(* Logix 5000 AddOnInstructionDefinition export NTEC_VerifyLimits; software revision ? *)

TYPE NTEC_Axis :   // NTEC Axis:
STRUCT
   StatDriveCommsOK : BOOL;   // Drive is communicating over ENET IP
   StatServoActionStatus : BOOL;   // Motion is enabled and holding position under power.
   StatDriveWarning : BOOL;   // Drive has a Warning
   StatDriveFault : BOOL;   // Drive is Faulted
   StatMotion_AtTarget : BOOL;   // Motion Target Reached
   StatMotion_FollowingError : BOOL;   // Following Error Fault
   StatMotion_LimitExceeded : BOOL;   // Speed or Position Limit Exceeded
   StatMotion_Halt : BOOL;   // Motor is in Halt, still powered on
   StatQuckStop : BOOL;   // Motor is powered off in Quick Stop
   StatMotion_Homed : BOOL;   // Motion Coordinate System Homed
   StatNewCmdToggle : BOOL;   // Bit toggles after new command accepted
   StatCommandError : BOOL;   // Last Command has an Error
   StatCommandErrorCode : DINT;   // Command Error Code
   StatDriveFaultCode : DINT;   // Drive Fault Code
   StatDriveWarningCode : DINT;   // Drive Warning Code
   StatResettingFault : BOOL;   // In fault reset sequence
   StatReadResponse : DINT;   // Response from a Read CMD
   CMD_IP : BOOL;   // Command is In Process
   CMD_DN : BOOL;   // Command is Done
   CMD_ERR : BOOL;   // Command Error during Comms send to Drive
   PDI_CMD : NTEC_PDI_CMD;   // Commands from AOIs
   PDI_Status : NTEC_PDI_Status;   // Status from Drive out to AOIs
   DriveLimits : NTEC_LimitsInDrive;   // Limits read from Drive
END_STRUCT
END_TYPE

TYPE NTEC_LimitsInDrive :   // These are the limits read from the Drive
STRUCT
   PositionLimitMin : DINT;   // Minimum Allowed Position Target (607Bh:1)
   PositionLimitMax : DINT;   // Maximum Allowed Position Target (607Bh:2)
   SoftPositionLimitMin : DINT;   // Minimum Allowed Position (607Dh:1)
   SoftPositionLimitMax : DINT;   // Minimum Allowed Position (607Dh:2)
   VelocityLimitMin : DINT;   // Maximum Allowed Velocity Target negative direction
   VelocityLimitMax : DINT;   // Maximum Allowed Velocity Target positive direction (607Fh)
   MotorSpeedMin : DINT;   // Maximum motor speed in negative direction
   MotorSpeedMax : DINT;   // Maximum motor speed setting in positive direction (6080h)
   AccelLimitMax : DINT;   // Maximum Allowed Accel Target (60C5h)
   DecelLimitMax : DINT;   // Maximum Allowed Decel Target (60C6h)
   PositionWindowNeg : DINT;   // Position Window - negative direction for At Target (6067h)
   PositionWindowPos : DINT;   // Position Window -positive direction for At Target (+/- this value) (6067h)
   VelocityWindowNeg : DINT;   // Velocity Window - negative side for At Target (+/- this value) (606Dh)
   VelocityWindowPos : DINT;   // Velocity Window - positive side for At Target (+/- this value) (606Dh)
   TorqueMaxNegDir : DINT;   // Maximum Torque Target negative direction (0.1% of motor rated current 2031h) (6072h)
   TorqueMaxPosDir : DINT;   // Maximum Torque Target positive direction (0.1% of motor rated current 2031h) (6072h)
   CurrentMaxNegDir : DINT;   // Maximum Current Target negative direction (in 0.1% of rated setting 2031h) (6073h)
   CurrentMaxPosDir : DINT;   // Maximum Current Target positive direction (in 0.1% of rated setting 2031h) (6073h)
END_STRUCT
END_TYPE

TYPE NTEC_PDI_CMD :   // PDI Command Bytes
STRUCT
   SetValue1 : DINT;
   SetValue2 : INT;
   SetValue3 : SINT;
   CMD : SINT;
   DigitalOutputs : DINT;
   NanoJ_Input1 : DINT;
   Trig : BOOL;   // Trigger the Command
   Halt : BOOL;   // Command a HALT
   QuickStop : BOOL;   // Command a QuickStop
END_STRUCT
END_TYPE

TYPE NTEC_PDI_Status :   // PDI Status Bytes
STRUCT
   Status : INT;
   ErrorCode : INT;
   ReturnValue : DINT;
   PositionActualValue : DINT;
   VelocityActualValue : DINT;
   DigitalInputs : DINT;
   TorqueActualValue : INT;
   AnalogInput1 : INT;
   FollowingError : DINT;
   NanoJ_Output1 : DINT;
END_STRUCT
END_TYPE

ADD_ON_INSTRUCTION NTEC_READ   (* revision 1.6, vendor Third Coast Automation, Nashville, TN, ExecutePrescan, ExecuteEnableInFalse *)
// READ instruction reads the value of  one object from the Drive.  Enter the target object's index and sub-index (typically 16#xxxx hex values).
// Revision note:
// Release Aug 27, 2024, update CPS instructions LEN
// Help:
// AOI written by:
// Tim Cochran
// Third Coast Automation
// Nashville, TN
// MAS ERR_Codes:
// 2: Input parameter range error – review and fix input parameters.
// 3: Command Error response from the Drive after command sent.
// 10: Communications Failed to Drive.
// 11: Drive Fault during this AOIs command sequence.
// 12: Quick Stop triggered by software outside of this AOI.
// 13: Command Error response from the Drive.
// 14: Enable input changed to False during sequence due to Drive Fault or Offline.
VAR_IN_OUT
   NTEC_Axis : NTEC_Axis; {required}   // NTEC Axis Tag
END_VAR
VAR_INPUT
   Index : DINT; {required}   // Index
   SubIndex : DINT; {required}   // Sub-Index
END_VAR
VAR_OUTPUT
   EN : BOOL; {visible}   // Enabled
   DN : BOOL; {visible}   // Successfully Done
   Read_Value : DINT; {visible}   // Value Read from Drive
   ERR : BOOL; {visible}   // Instruction Error
   ERR_Code : DINT; {access Read Only, visible}   // Instruction Error Code
END_VAR
VAR
   State : DINT; {access None}
   Enable : BOOL; {access None}
   InputRangesOK : BOOL; {access None}
   local_SubIndex : DINT; {access None}
   local_Index : DINT; {access None}
   tmr_Verify : TIMER := (PRE := 20); {access None}
END_VAR

ROUTINE EnableInFalse   (* ladder *)
// Enable In False Routine
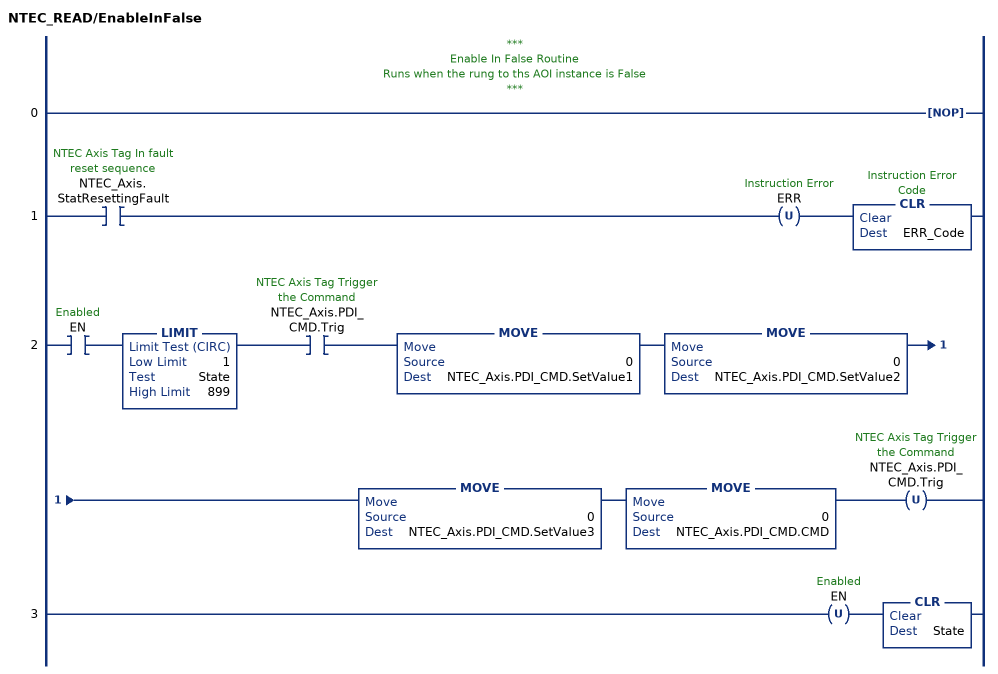
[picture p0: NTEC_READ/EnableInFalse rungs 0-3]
   // ***
   // Enable In False Routine
   // Runs when the rung to ths AOI instance is False
   // ***
   0: NOP();
   1: XIC(NTEC_Axis.StatResettingFault)OTU(ERR)CLR(ERR_Code);
   2: XIC(EN)LIMIT(1,State,899)XIC(NTEC_Axis.PDI_CMD.Trig)MOVE(0,NTEC_Axis.PDI_CMD.SetValue1)MOVE(0,NTEC_Axis.PDI_CMD.SetValue2)MOVE(0,NTEC_Axis.PDI_CMD.SetValue3)MOVE(0,NTEC_Axis.PDI_CMD.CMD)OTU(NTEC_Axis.PDI_CMD.Trig);
   3: OTU(EN)CLR(State);
END_ROUTINE

ROUTINE Logic   (* ladder *)
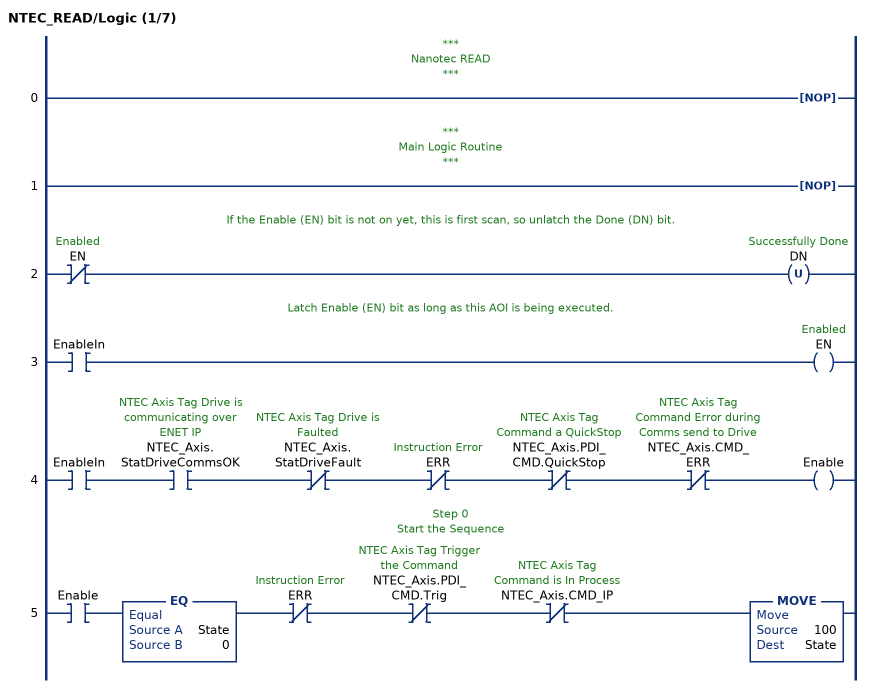
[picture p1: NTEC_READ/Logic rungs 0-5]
   // ***
   // Nanotec READ
   // ***
   0: NOP();
   // ***
   // Main Logic Routine
   // ***
   1: NOP();
   // If the Enable (EN) bit is not on yet, this is first scan, so unlatch the Done (DN) bit.
   2: XIO(EN)OTU(DN);
   // Latch Enable (EN) bit as long as this AOI is being executed.
   3: XIC(EnableIn)OTE(EN);
   4: XIC(EnableIn)XIC(NTEC_Axis.StatDriveCommsOK)XIO(NTEC_Axis.StatDriveFault)XIO(ERR)XIO(NTEC_Axis.PDI_CMD.QuickStop)XIO(NTEC_Axis.CMD_ERR)OTE(Enable);
   // Step 0
   // Start the Sequence
   5: XIC(Enable)EQ(State,0)XIO(ERR)XIO(NTEC_Axis.PDI_CMD.Trig)XIO(NTEC_Axis.CMD_IP)MOVE(100,State);
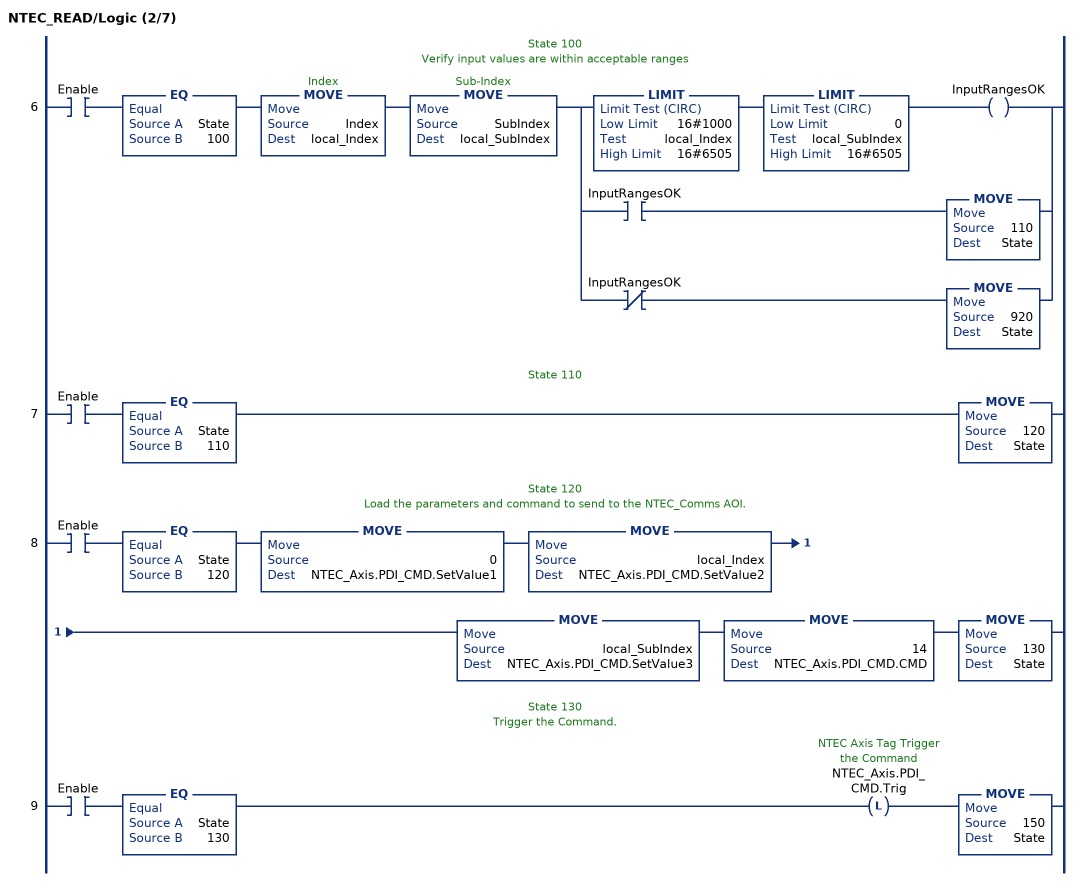
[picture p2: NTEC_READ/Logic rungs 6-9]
   // State 100
   // Verify input values are within acceptable ranges
   6: XIC(Enable)EQ(State,100)MOVE(Index,local_Index)MOVE(SubIndex,local_SubIndex)[LIMIT(16#1000,local_Index,16#6505) LIMIT(0,local_SubIndex,16#6505) OTE(InputRangesOK) ,XIC(InputRangesOK) MOVE(110,State) ,XIO(InputRangesOK) MOVE(920,State) ];
   // State 110
   7: XIC(Enable)EQ(State,110)MOVE(120,State);
   // State 120
   // Load the parameters and command to send to the NTEC_Comms AOI.
   8: XIC(Enable)EQ(State,120)MOVE(0,NTEC_Axis.PDI_CMD.SetValue1)MOVE(local_Index,NTEC_Axis.PDI_CMD.SetValue2)MOVE(local_SubIndex,NTEC_Axis.PDI_CMD.SetValue3)MOVE(14,NTEC_Axis.PDI_CMD.CMD)MOVE(130,State);
   // State 130
   // Trigger the Command.
   9: XIC(Enable)EQ(State,130)OTL(NTEC_Axis.PDI_CMD.Trig)MOVE(150,State);
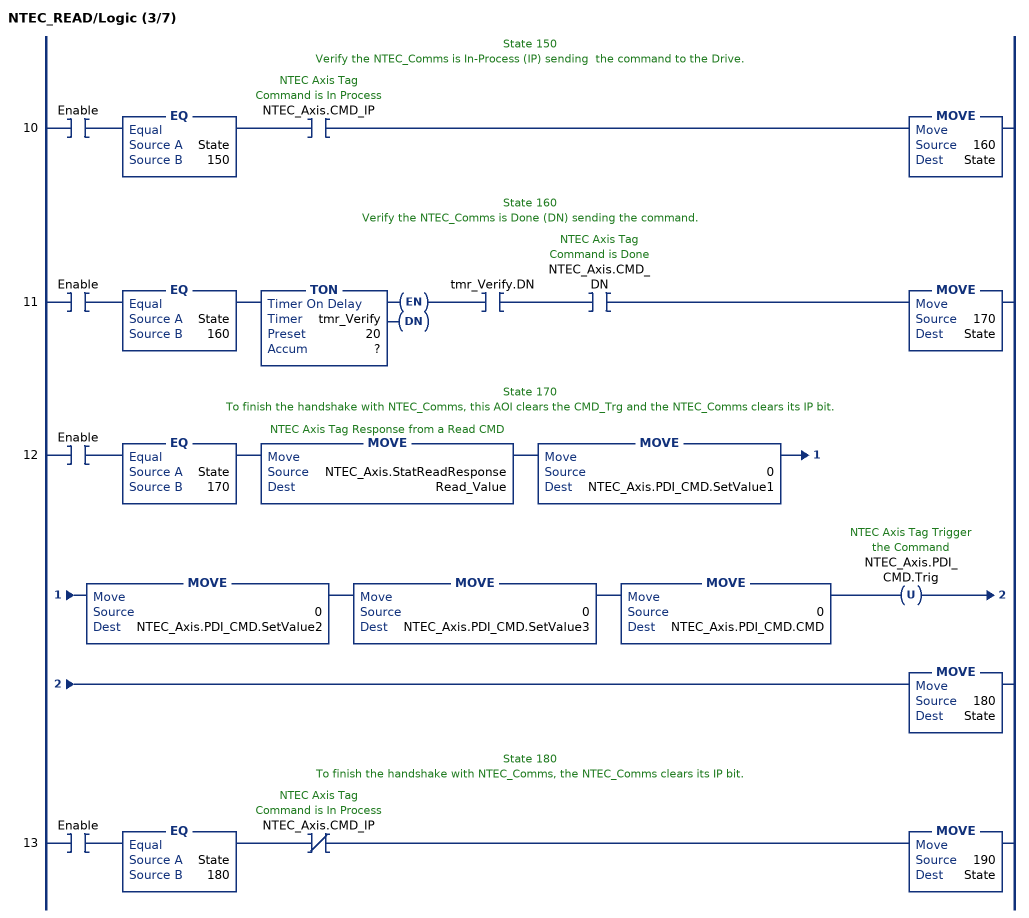
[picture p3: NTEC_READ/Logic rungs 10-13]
   // State 150
   // Verify the NTEC_Comms is In-Process (IP) sending  the command to the Drive.
   10: XIC(Enable)EQ(State,150)XIC(NTEC_Axis.CMD_IP)MOVE(160,State);
   // State 160
   // Verify the NTEC_Comms is Done (DN) sending the command.
   11: XIC(Enable)EQ(State,160)TON(tmr_Verify,?,?)XIC(tmr_Verify.DN)XIC(NTEC_Axis.CMD_DN)MOVE(170,State);
   // State 170
   // To finish the handshake with NTEC_Comms, this AOI clears the CMD_Trg and the NTEC_Comms clears its IP bit.
   12: XIC(Enable)EQ(State,170)MOVE(NTEC_Axis.StatReadResponse,Read_Value)MOVE(0,NTEC_Axis.PDI_CMD.SetValue1)MOVE(0,NTEC_Axis.PDI_CMD.SetValue2)MOVE(0,NTEC_Axis.PDI_CMD.SetValue3)MOVE(0,NTEC_Axis.PDI_CMD.CMD)OTU(NTEC_Axis.PDI_CMD.Trig)MOVE(180,State);
   // State 180
   // To finish the handshake with NTEC_Comms, the NTEC_Comms clears its IP bit.
   13: XIC(Enable)EQ(State,180)XIO(NTEC_Axis.CMD_IP)MOVE(190,State);
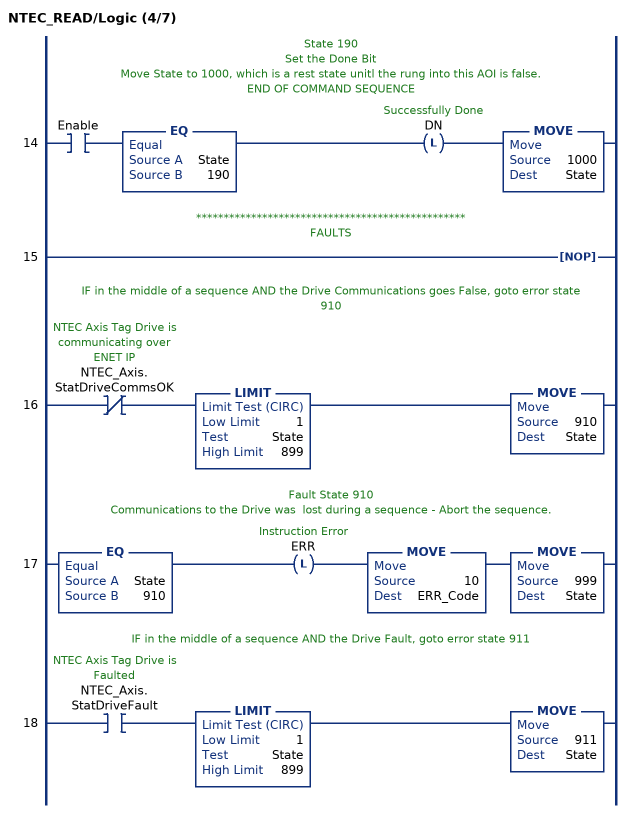
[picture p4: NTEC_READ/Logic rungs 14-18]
   // State 190
   // Set the Done Bit
   // Move State to 1000, which is a rest state unitl the rung into this AOI is false.
   // END OF COMMAND SEQUENCE
   14: XIC(Enable)EQ(State,190)OTL(DN)MOVE(1000,State);
   // *************************************************
   // FAULTS
   15: NOP();
   // IF in the middle of a sequence AND the Drive Communications goes False, goto error state 910
   16: XIO(NTEC_Axis.StatDriveCommsOK)LIMIT(1,State,899)MOVE(910,State);
   // Fault State 910
   // Communications to the Drive was  lost during a sequence - Abort the sequence.
   17: EQ(State,910)OTL(ERR)MOVE(10,ERR_Code)MOVE(999,State);
   // IF in the middle of a sequence AND the Drive Fault, goto error state 911
   18: XIC(NTEC_Axis.StatDriveFault)LIMIT(1,State,899)MOVE(911,State);
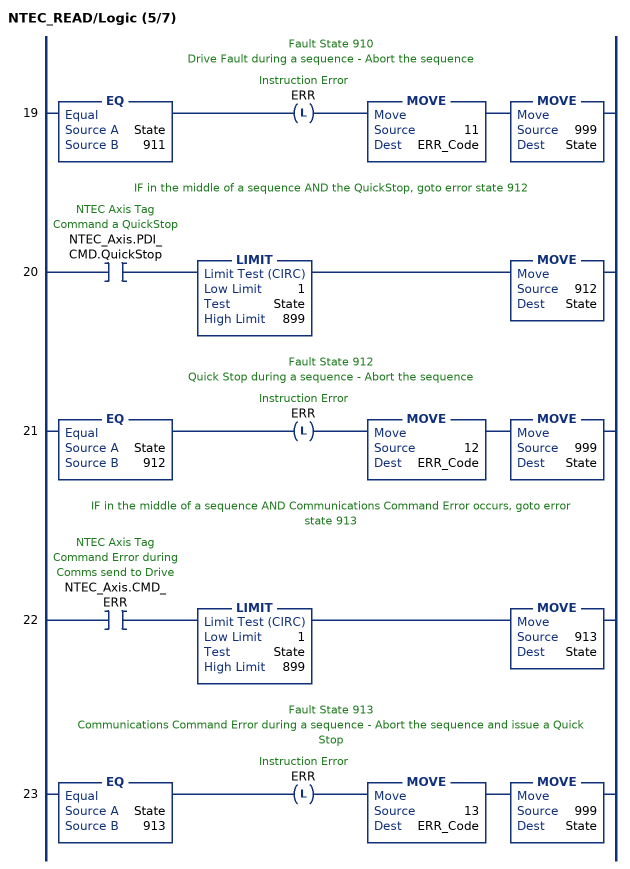
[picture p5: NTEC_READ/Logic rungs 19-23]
   // Fault State 910
   // Drive Fault during a sequence - Abort the sequence
   19: EQ(State,911)OTL(ERR)MOVE(11,ERR_Code)MOVE(999,State);
   // IF in the middle of a sequence AND the QuickStop, goto error state 912
   20: XIC(NTEC_Axis.PDI_CMD.QuickStop)LIMIT(1,State,899)MOVE(912,State);
   // Fault State 912
   // Quick Stop during a sequence - Abort the sequence
   21: EQ(State,912)OTL(ERR)MOVE(12,ERR_Code)MOVE(999,State);
   // IF in the middle of a sequence AND Communications Command Error occurs, goto error state 913
   22: XIC(NTEC_Axis.CMD_ERR)LIMIT(1,State,899)MOVE(913,State);
   // Fault State 913
   // Communications Command Error during a sequence - Abort the sequence and issue a Quick Stop
   23: EQ(State,913)OTL(ERR)MOVE(13,ERR_Code)MOVE(999,State);
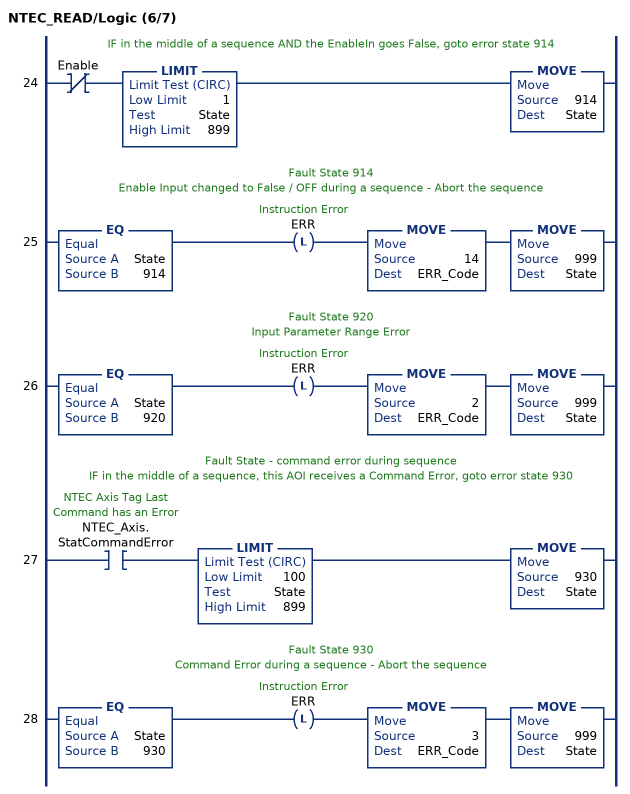
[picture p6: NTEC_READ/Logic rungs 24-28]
   // IF in the middle of a sequence AND the EnableIn goes False, goto error state 914
   24: XIO(Enable)LIMIT(1,State,899)MOVE(914,State);
   // Fault State 914
   // Enable Input changed to False / OFF during a sequence - Abort the sequence
   25: EQ(State,914)OTL(ERR)MOVE(14,ERR_Code)MOVE(999,State);
   // Fault State 920
   // Input Parameter Range Error
   26: EQ(State,920)OTL(ERR)MOVE(2,ERR_Code)MOVE(999,State);
   // Fault State - command error during sequence
   // IF in the middle of a sequence, this AOI receives a Command Error, goto error state 930
   27: XIC(NTEC_Axis.StatCommandError)LIMIT(100,State,899)MOVE(930,State);
   // Fault State 930
   // Command Error during a sequence - Abort the sequence
   28: EQ(State,930)OTL(ERR)MOVE(3,ERR_Code)MOVE(999,State);
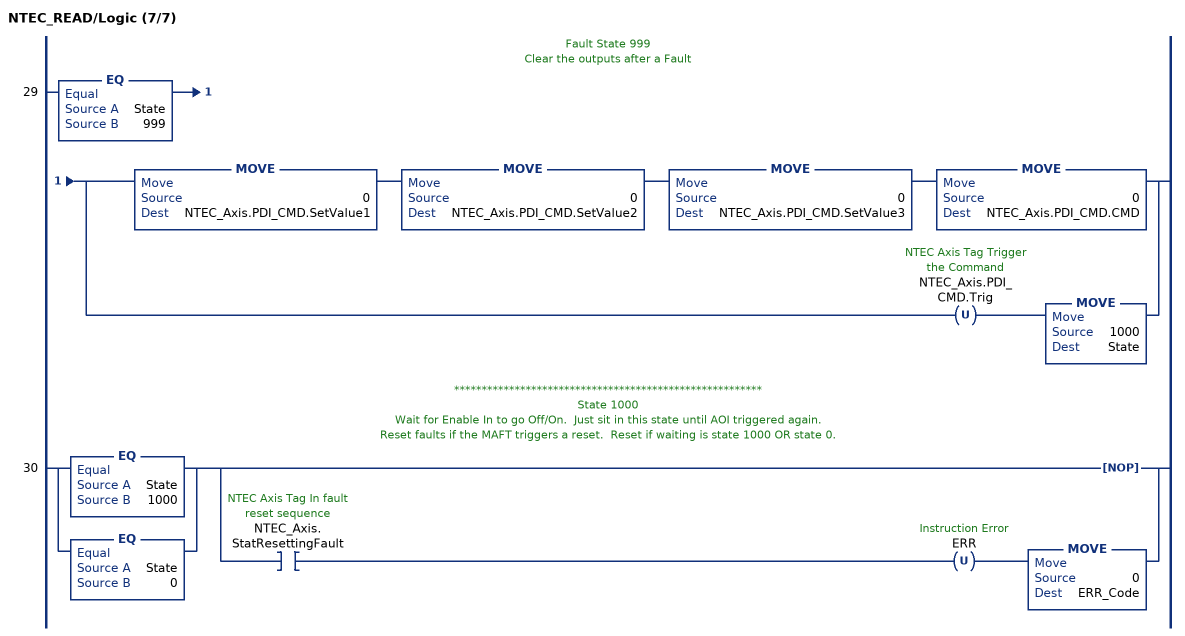
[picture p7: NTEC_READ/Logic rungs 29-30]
   // Fault State 999
   // Clear the outputs after a Fault
   29: EQ(State,999)[MOVE(0,NTEC_Axis.PDI_CMD.SetValue1) MOVE(0,NTEC_Axis.PDI_CMD.SetValue2) MOVE(0,NTEC_Axis.PDI_CMD.SetValue3) MOVE(0,NTEC_Axis.PDI_CMD.CMD) ,OTU(NTEC_Axis.PDI_CMD.Trig) MOVE(1000,State) ];
   // ********************************************************
   // State 1000
   // Wait for Enable In to go Off/On.  Just sit in this state until AOI triggered again.
   // Reset faults if the MAFT triggers a reset.  Reset if waiting is state 1000 OR state 0.
   30: [EQ(State,1000) ,EQ(State,0) ][NOP() ,XIC(NTEC_Axis.StatResettingFault) OTU(ERR) MOVE(0,ERR_Code) ];
END_ROUTINE

ROUTINE Postscan   (* ladder *)
// Home Post-Scan Routine
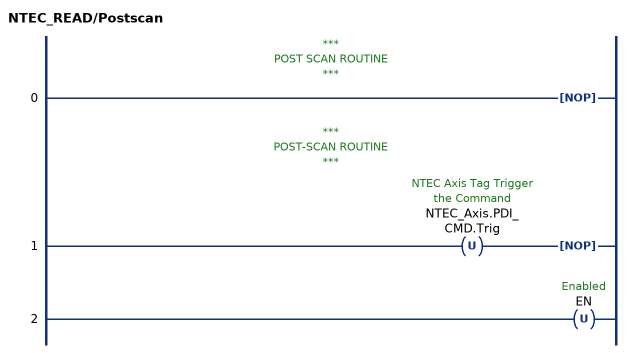
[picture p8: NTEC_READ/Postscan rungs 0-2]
   // ***
   // POST SCAN ROUTINE
   // ***
   0: NOP();
   // ***
   // POST-SCAN ROUTINE
   // ***
   1: OTU(NTEC_Axis.PDI_CMD.Trig)NOP();
   2: OTU(EN);
END_ROUTINE

ROUTINE Prescan   (* ladder *)
// Home Pre-Scan Routine
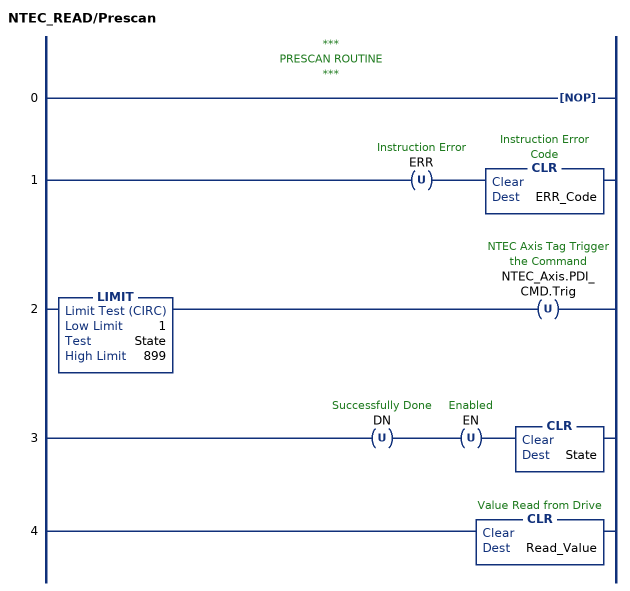
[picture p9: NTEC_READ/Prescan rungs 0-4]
   // ***
   // PRESCAN ROUTINE
   // ***
   0: NOP();
   1: OTU(ERR)CLR(ERR_Code);
   2: LIMIT(1,State,899)OTU(NTEC_Axis.PDI_CMD.Trig);
   3: OTU(DN)OTU(EN)CLR(State);
   4: CLR(Read_Value);
END_ROUTINE
END_ADD_ON_INSTRUCTION

ADD_ON_INSTRUCTION NTEC_VerifyLimits   (* revision 1.6, vendor Third Coast Automation, Nashville, TN, ExecutePrescan, ExecuteEnableInFalse *)
// This AOI is only used in the COMMS AOI.
// Only at the first scan of the COMMS AOI, this AOI is called to read all of the limit values from theDrive.  Limits are used to check AOI input values.
// Revision note:
// Release Aug 27, 2024, update CPS instructions LEN
// Help:
// AOI written by:
// Tim Cochran
// Third Coast Automation
// Nashville, TN
// VerifyLimits ERR_Codes:
// 2: Input parameter range error – review and fix input parameters.
// 3: Command Error response from the Drive after command sent.
// 10: Communications Failed to Drive.
// 11: Drive Fault during this AOIs command sequence.
// 12: Quick Stop triggered by software outside of this AOI.
// 13: Command Error response from the Drive.
// 14: Enable input changed to False during sequence due to Drive Fault or Offline.
// 610: Error trying to read the Position Range Limit Minimum (607Bh:1) value from the Drive.
// 630: Error trying to read the Position Range Limit Maximum (607Bh:2) value from the Drive.
// 650: Error trying to read the Software Position Range Limit Minimum (607Dh:1) value from the Drive.
// 670: Error trying to read the Software Position Range Limit Maximum (607Dh:2) value from the Drive.
// 690: Error trying to read the Velocity Limit (607Fh:0) value from the Drive.
// 710: Error trying to read the Max Motor Speed (6080h:0) value from the Drive.
// 730: Error trying to read the Acceleration Limit (60C5h:0) value from the Drive.
// 750: Error trying to read the Deceleration Limit (60C6h:0) value from the Drive.
// 770: Error trying to read the Position Window (6067h:0) value from the Drive.
// 790: Error trying to read the Velocity Window (606Dh:0) value from the Drive.
// 810: Error trying to read the Max Torque Limit (6072h:0) value from the Drive.
// 810: Error trying to read the Max Current Limit (6073h:0) value from the Drive.
VAR_IN_OUT
   NTEC_Axis : NTEC_Axis; {required}   // NTEC Axis Tag
END_VAR
VAR_OUTPUT
   EN : BOOL; {visible}   // Enabled
   DN : BOOL; {visible}   // Successfully Done
   ERR : BOOL; {visible}   // Instruction Error
   ERR_Code : DINT; {access Read Only, visible}   // Instruction Error Code
END_VAR
VAR
   State : DINT; {access None}
   Enable : BOOL; {access None}
   InputRangesOK : BOOL; {access None}
   cntrl_ReadLimits1 : NTEC_READ; {access None}
   cntrl_ReadLimits2 : NTEC_READ; {access None}
   cntrl_ReadLimits3 : NTEC_READ; {access None}
   cntrl_ReadLimits4 : NTEC_READ; {access None}
   cntrl_ReadLimits5 : NTEC_READ; {access None}
   cntrl_ReadLimits6 : NTEC_READ; {access None}
   cntrl_ReadLimits7 : NTEC_READ; {access None}
   cntrl_ReadLimits8 : NTEC_READ; {access None}
   cntrl_ReadLimits9 : NTEC_READ; {access None}
   cntrl_ReadLimits10 : NTEC_READ; {access None}
   cntrl_ReadLimits11 : NTEC_READ; {access None}
   cntrl_ReadLimits12 : NTEC_READ; {access None}
END_VAR

ROUTINE EnableInFalse   (* ladder *)
// Enable In False Routine
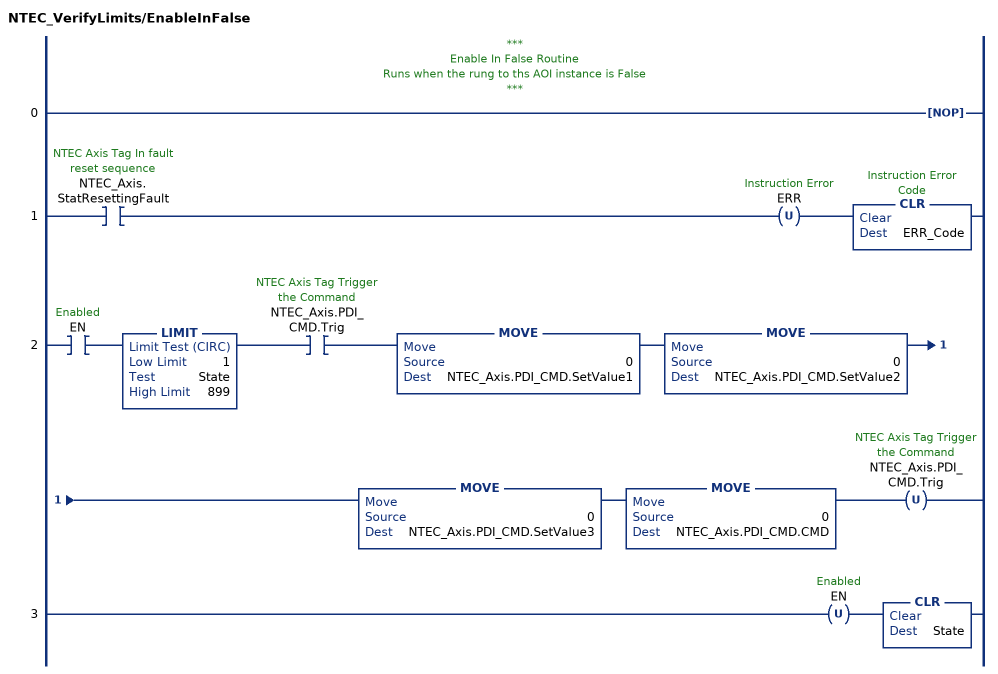
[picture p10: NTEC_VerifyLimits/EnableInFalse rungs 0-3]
   // ***
   // Enable In False Routine
   // Runs when the rung to ths AOI instance is False
   // ***
   0: NOP();
   1: XIC(NTEC_Axis.StatResettingFault)OTU(ERR)CLR(ERR_Code);
   2: XIC(EN)LIMIT(1,State,899)XIC(NTEC_Axis.PDI_CMD.Trig)MOVE(0,NTEC_Axis.PDI_CMD.SetValue1)MOVE(0,NTEC_Axis.PDI_CMD.SetValue2)MOVE(0,NTEC_Axis.PDI_CMD.SetValue3)MOVE(0,NTEC_Axis.PDI_CMD.CMD)OTU(NTEC_Axis.PDI_CMD.Trig);
   3: OTU(EN)CLR(State);
END_ROUTINE

ROUTINE Logic   (* ladder *)
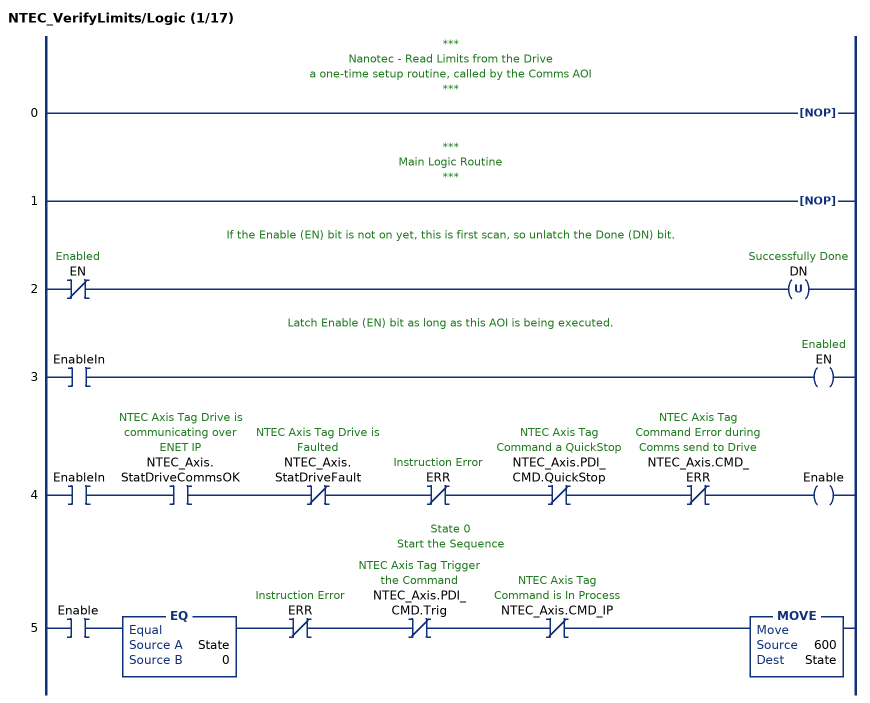
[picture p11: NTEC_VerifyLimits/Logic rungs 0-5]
   // ***
   // Nanotec - Read Limits from the Drive
   // a one-time setup routine, called by the Comms AOI
   // ***
   0: NOP();
   // ***
   // Main Logic Routine
   // ***
   1: NOP();
   // If the Enable (EN) bit is not on yet, this is first scan, so unlatch the Done (DN) bit.
   2: XIO(EN)OTU(DN);
   // Latch Enable (EN) bit as long as this AOI is being executed.
   3: XIC(EnableIn)OTE(EN);
   4: XIC(EnableIn)XIC(NTEC_Axis.StatDriveCommsOK)XIO(NTEC_Axis.StatDriveFault)XIO(ERR)XIO(NTEC_Axis.PDI_CMD.QuickStop)XIO(NTEC_Axis.CMD_ERR)OTE(Enable);
   // State 0
   // Start the Sequence
   5: XIC(Enable)EQ(State,0)XIO(ERR)XIO(NTEC_Axis.PDI_CMD.Trig)XIO(NTEC_Axis.CMD_IP)MOVE(600,State);
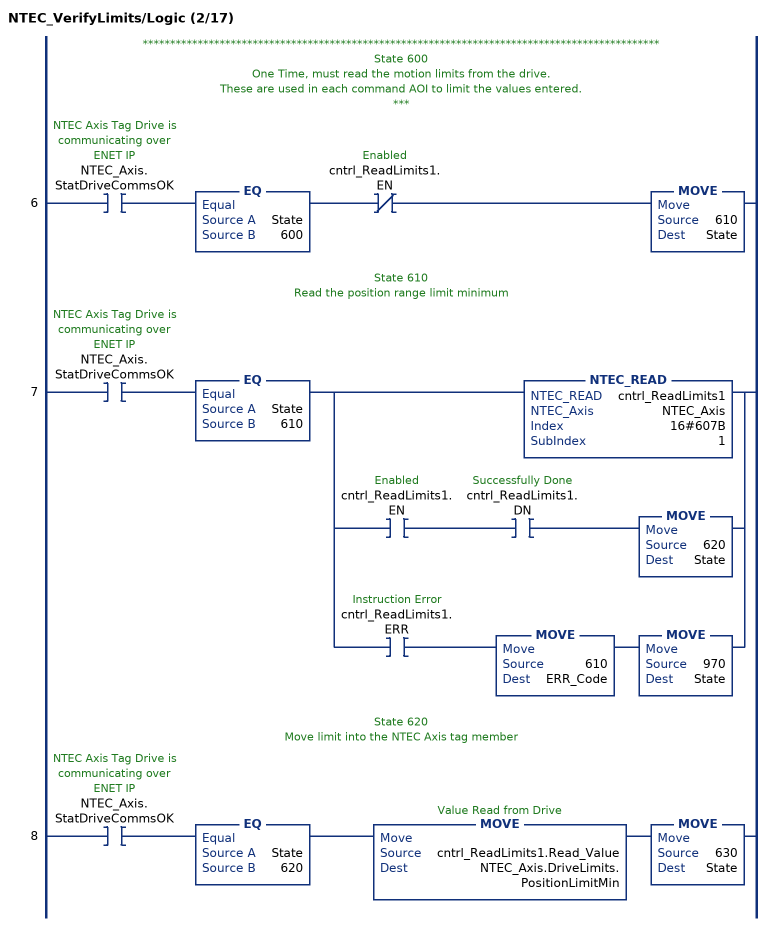
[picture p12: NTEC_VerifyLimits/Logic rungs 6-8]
   // **********************************************************************************************
   // State 600
   // One Time, must read the motion limits from the drive.
   // These are used in each command AOI to limit the values entered.
   //  ***
   6: XIC(NTEC_Axis.StatDriveCommsOK)EQ(State,600)XIO(cntrl_ReadLimits1.EN)MOVE(610,State);
   // State 610
   //   Read the position range limit minimum
   7: XIC(NTEC_Axis.StatDriveCommsOK)EQ(State,610)[NTEC_READ(cntrl_ReadLimits1,NTEC_Axis,16#607B,1) ,XIC(cntrl_ReadLimits1.EN) XIC(cntrl_ReadLimits1.DN) MOVE(620,State) ,XIC(cntrl_ReadLimits1.ERR) MOVE(610,ERR_Code) MOVE(970,State) ];
   // State 620
   // Move limit into the NTEC Axis tag member
   8: XIC(NTEC_Axis.StatDriveCommsOK)EQ(State,620)MOVE(cntrl_ReadLimits1.Read_Value,NTEC_Axis.DriveLimits.PositionLimitMin)MOVE(630,State);
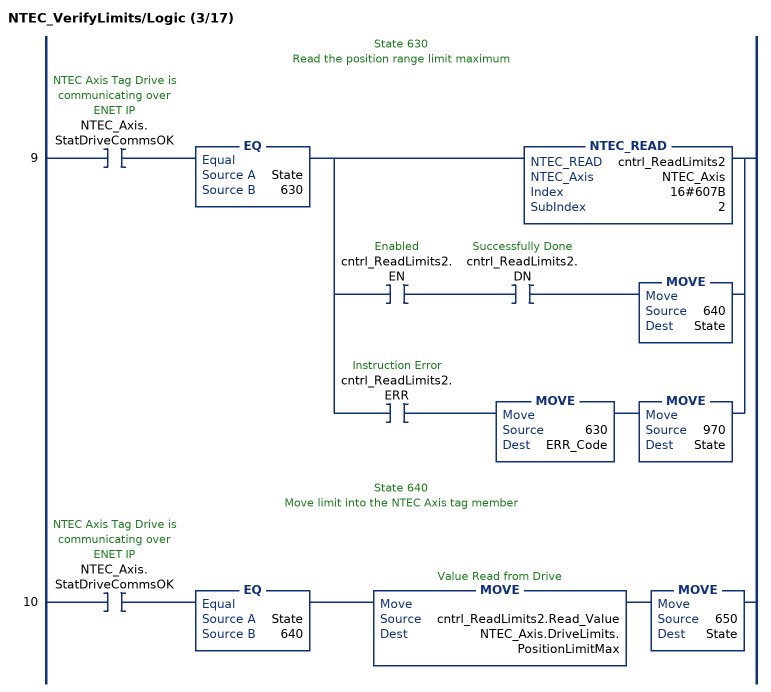
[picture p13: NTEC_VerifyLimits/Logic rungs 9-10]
   // State 630
   //   Read the position range limit maximum
   9: XIC(NTEC_Axis.StatDriveCommsOK)EQ(State,630)[NTEC_READ(cntrl_ReadLimits2,NTEC_Axis,16#607B,2) ,XIC(cntrl_ReadLimits2.EN) XIC(cntrl_ReadLimits2.DN) MOVE(640,State) ,XIC(cntrl_ReadLimits2.ERR) MOVE(630,ERR_Code) MOVE(970,State) ];
   // State 640
   // Move limit into the NTEC Axis tag member
   10: XIC(NTEC_Axis.StatDriveCommsOK)EQ(State,640)MOVE(cntrl_ReadLimits2.Read_Value,NTEC_Axis.DriveLimits.PositionLimitMax)MOVE(650,State);
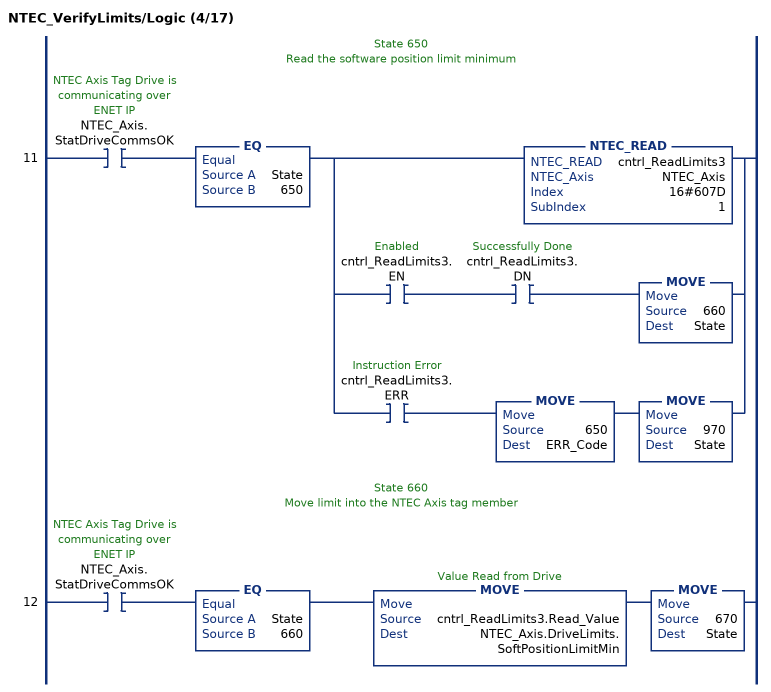
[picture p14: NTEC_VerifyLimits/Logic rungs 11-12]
   // State 650
   //   Read the software position limit minimum
   11: XIC(NTEC_Axis.StatDriveCommsOK)EQ(State,650)[NTEC_READ(cntrl_ReadLimits3,NTEC_Axis,16#607D,1) ,XIC(cntrl_ReadLimits3.EN) XIC(cntrl_ReadLimits3.DN) MOVE(660,State) ,XIC(cntrl_ReadLimits3.ERR) MOVE(650,ERR_Code) MOVE(970,State) ];
   // State 660
   // Move limit into the NTEC Axis tag member
   12: XIC(NTEC_Axis.StatDriveCommsOK)EQ(State,660)MOVE(cntrl_ReadLimits3.Read_Value,NTEC_Axis.DriveLimits.SoftPositionLimitMin)MOVE(670,State);
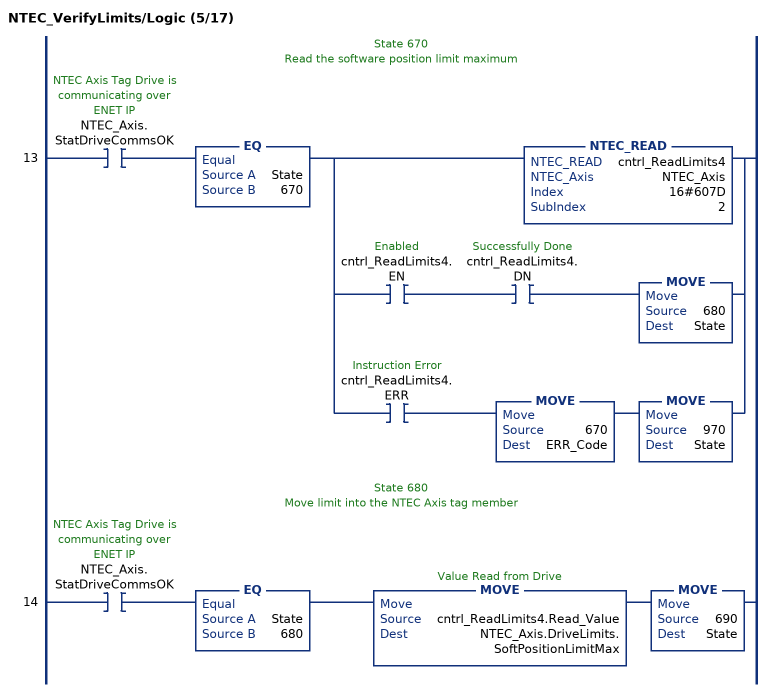
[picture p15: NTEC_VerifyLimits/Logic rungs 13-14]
   // State 670
   //   Read the software position limit maximum
   13: XIC(NTEC_Axis.StatDriveCommsOK)EQ(State,670)[NTEC_READ(cntrl_ReadLimits4,NTEC_Axis,16#607D,2) ,XIC(cntrl_ReadLimits4.EN) XIC(cntrl_ReadLimits4.DN) MOVE(680,State) ,XIC(cntrl_ReadLimits4.ERR) MOVE(670,ERR_Code) MOVE(970,State) ];
   // State 680
   // Move limit into the NTEC Axis tag member
   14: XIC(NTEC_Axis.StatDriveCommsOK)EQ(State,680)MOVE(cntrl_ReadLimits4.Read_Value,NTEC_Axis.DriveLimits.SoftPositionLimitMax)MOVE(690,State);
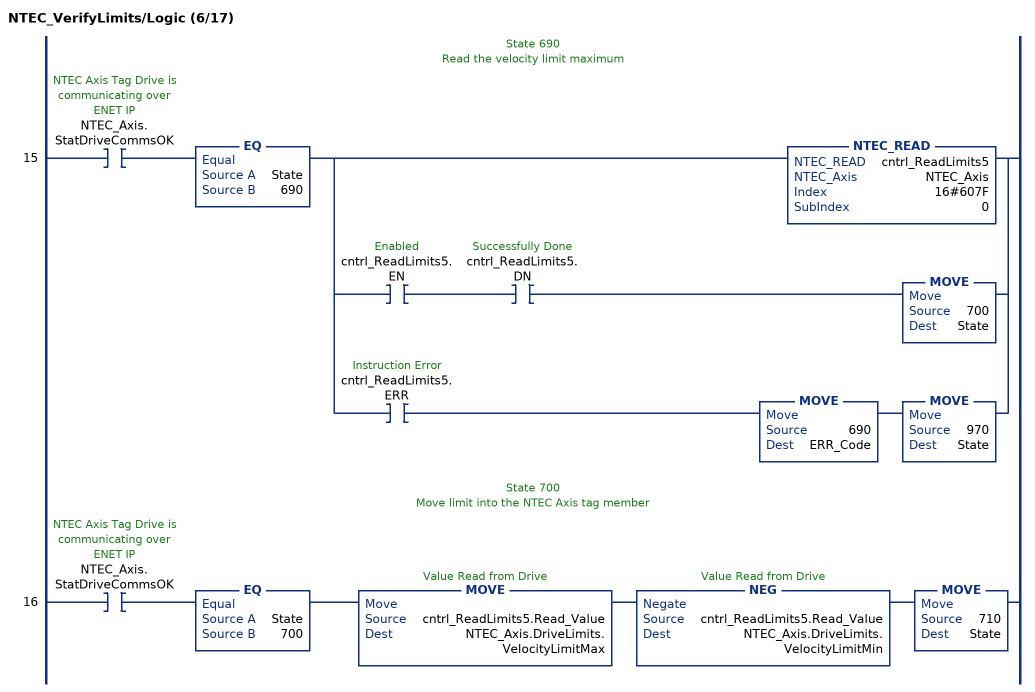
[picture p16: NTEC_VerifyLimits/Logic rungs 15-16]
   // State 690
   //   Read the velocity limit maximum
   15: XIC(NTEC_Axis.StatDriveCommsOK)EQ(State,690)[NTEC_READ(cntrl_ReadLimits5,NTEC_Axis,16#607F,0) ,XIC(cntrl_ReadLimits5.EN) XIC(cntrl_ReadLimits5.DN) MOVE(700,State) ,XIC(cntrl_ReadLimits5.ERR) MOVE(690,ERR_Code) MOVE(970,State) ];
   // State 700
   // Move limit into the NTEC Axis tag member
   16: XIC(NTEC_Axis.StatDriveCommsOK)EQ(State,700)MOVE(cntrl_ReadLimits5.Read_Value,NTEC_Axis.DriveLimits.VelocityLimitMax)NEG(cntrl_ReadLimits5.Read_Value,NTEC_Axis.DriveLimits.VelocityLimitMin)MOVE(710,State);
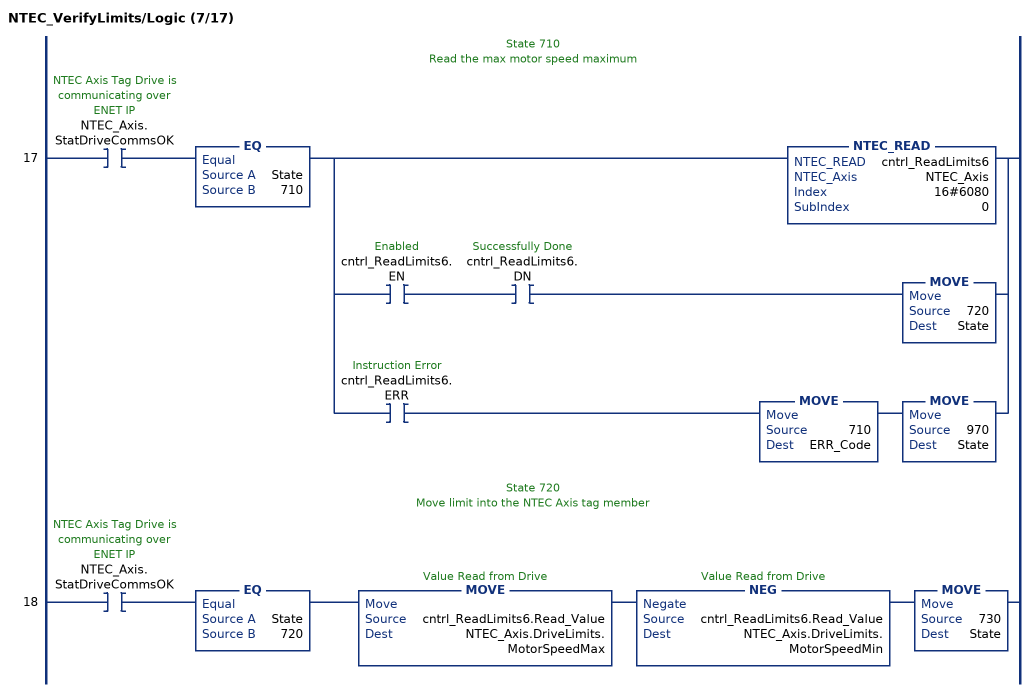
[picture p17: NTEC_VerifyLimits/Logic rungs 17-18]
   // State 710
   //   Read the max motor speed maximum
   17: XIC(NTEC_Axis.StatDriveCommsOK)EQ(State,710)[NTEC_READ(cntrl_ReadLimits6,NTEC_Axis,16#6080,0) ,XIC(cntrl_ReadLimits6.EN) XIC(cntrl_ReadLimits6.DN) MOVE(720,State) ,XIC(cntrl_ReadLimits6.ERR) MOVE(710,ERR_Code) MOVE(970,State) ];
   // State 720
   // Move limit into the NTEC Axis tag member
   18: XIC(NTEC_Axis.StatDriveCommsOK)EQ(State,720)MOVE(cntrl_ReadLimits6.Read_Value,NTEC_Axis.DriveLimits.MotorSpeedMax)NEG(cntrl_ReadLimits6.Read_Value,NTEC_Axis.DriveLimits.MotorSpeedMin)MOVE(730,State);
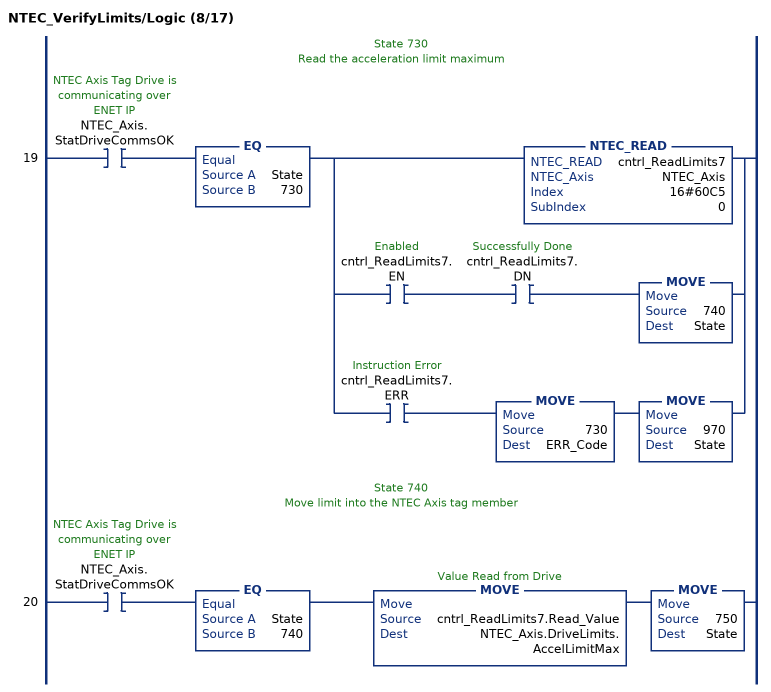
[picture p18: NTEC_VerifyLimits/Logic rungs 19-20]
   // State 730
   //   Read the acceleration limit maximum
   19: XIC(NTEC_Axis.StatDriveCommsOK)EQ(State,730)[NTEC_READ(cntrl_ReadLimits7,NTEC_Axis,16#60C5,0) ,XIC(cntrl_ReadLimits7.EN) XIC(cntrl_ReadLimits7.DN) MOVE(740,State) ,XIC(cntrl_ReadLimits7.ERR) MOVE(730,ERR_Code) MOVE(970,State) ];
   // State 740
   // Move limit into the NTEC Axis tag member
   20: XIC(NTEC_Axis.StatDriveCommsOK)EQ(State,740)MOVE(cntrl_ReadLimits7.Read_Value,NTEC_Axis.DriveLimits.AccelLimitMax)MOVE(750,State);
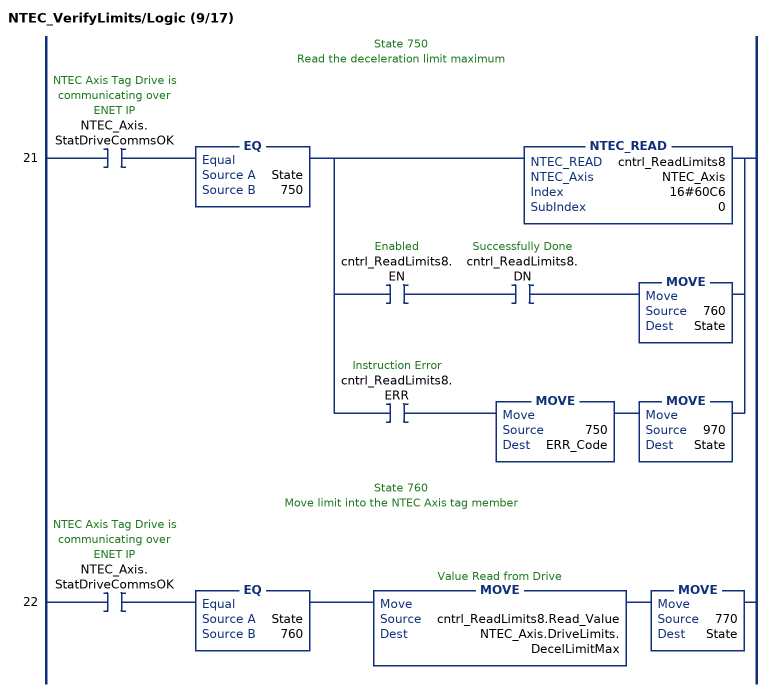
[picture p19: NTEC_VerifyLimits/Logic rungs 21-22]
   // State 750
   //   Read the deceleration limit maximum
   21: XIC(NTEC_Axis.StatDriveCommsOK)EQ(State,750)[NTEC_READ(cntrl_ReadLimits8,NTEC_Axis,16#60C6,0) ,XIC(cntrl_ReadLimits8.EN) XIC(cntrl_ReadLimits8.DN) MOVE(760,State) ,XIC(cntrl_ReadLimits8.ERR) MOVE(750,ERR_Code) MOVE(970,State) ];
   // State 760
   // Move limit into the NTEC Axis tag member
   22: XIC(NTEC_Axis.StatDriveCommsOK)EQ(State,760)MOVE(cntrl_ReadLimits8.Read_Value,NTEC_Axis.DriveLimits.DecelLimitMax)MOVE(770,State);
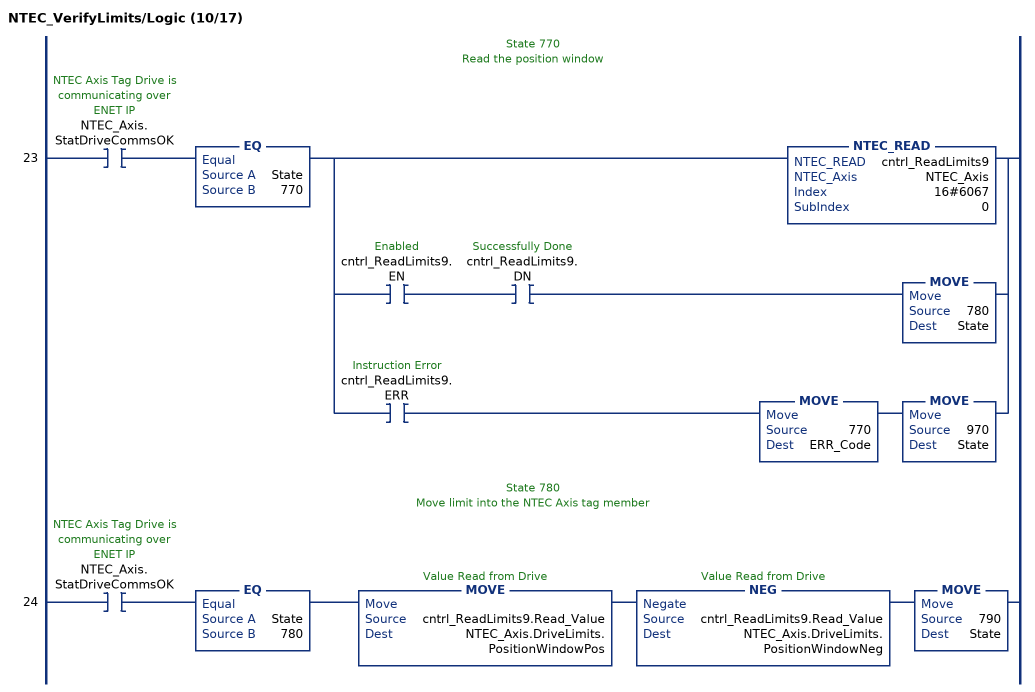
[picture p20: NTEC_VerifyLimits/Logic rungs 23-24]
   // State 770
   //   Read the position window
   23: XIC(NTEC_Axis.StatDriveCommsOK)EQ(State,770)[NTEC_READ(cntrl_ReadLimits9,NTEC_Axis,16#6067,0) ,XIC(cntrl_ReadLimits9.EN) XIC(cntrl_ReadLimits9.DN) MOVE(780,State) ,XIC(cntrl_ReadLimits9.ERR) MOVE(770,ERR_Code) MOVE(970,State) ];
   // State 780
   // Move limit into the NTEC Axis tag member
   24: XIC(NTEC_Axis.StatDriveCommsOK)EQ(State,780)MOVE(cntrl_ReadLimits9.Read_Value,NTEC_Axis.DriveLimits.PositionWindowPos)NEG(cntrl_ReadLimits9.Read_Value,NTEC_Axis.DriveLimits.PositionWindowNeg)MOVE(790,State);
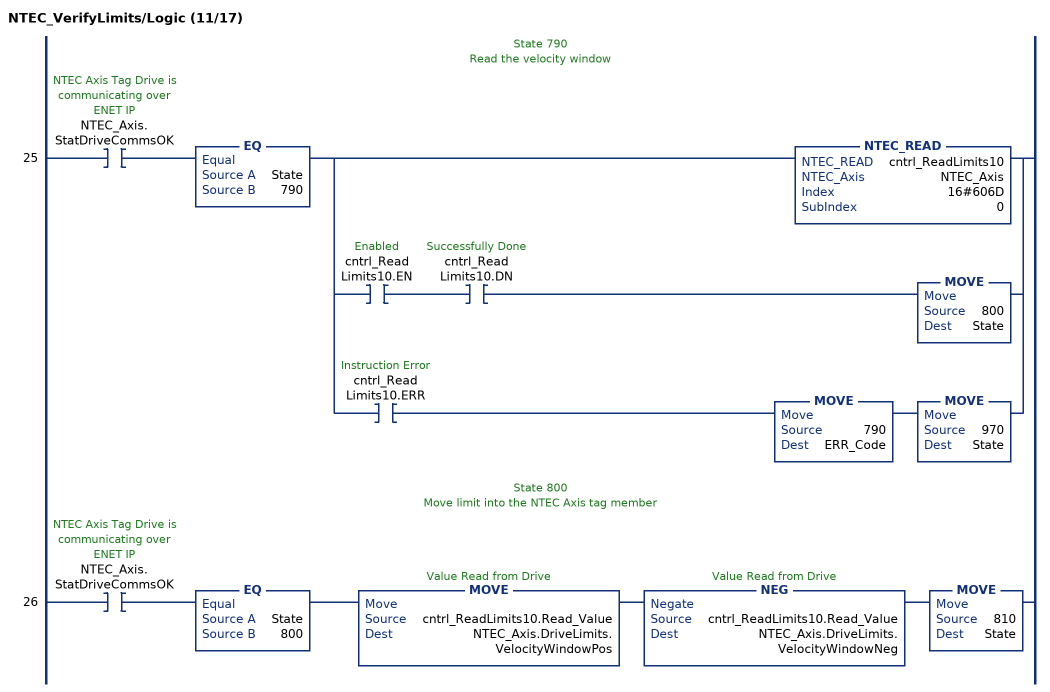
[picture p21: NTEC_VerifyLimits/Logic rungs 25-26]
   // State 790
   //   Read the velocity window
   25: XIC(NTEC_Axis.StatDriveCommsOK)EQ(State,790)[NTEC_READ(cntrl_ReadLimits10,NTEC_Axis,16#606D,0) ,XIC(cntrl_ReadLimits10.EN) XIC(cntrl_ReadLimits10.DN) MOVE(800,State) ,XIC(cntrl_ReadLimits10.ERR) MOVE(790,ERR_Code) MOVE(970,State) ];
   // State 800
   // Move limit into the NTEC Axis tag member
   26: XIC(NTEC_Axis.StatDriveCommsOK)EQ(State,800)MOVE(cntrl_ReadLimits10.Read_Value,NTEC_Axis.DriveLimits.VelocityWindowPos)NEG(cntrl_ReadLimits10.Read_Value,NTEC_Axis.DriveLimits.VelocityWindowNeg)MOVE(810,State);
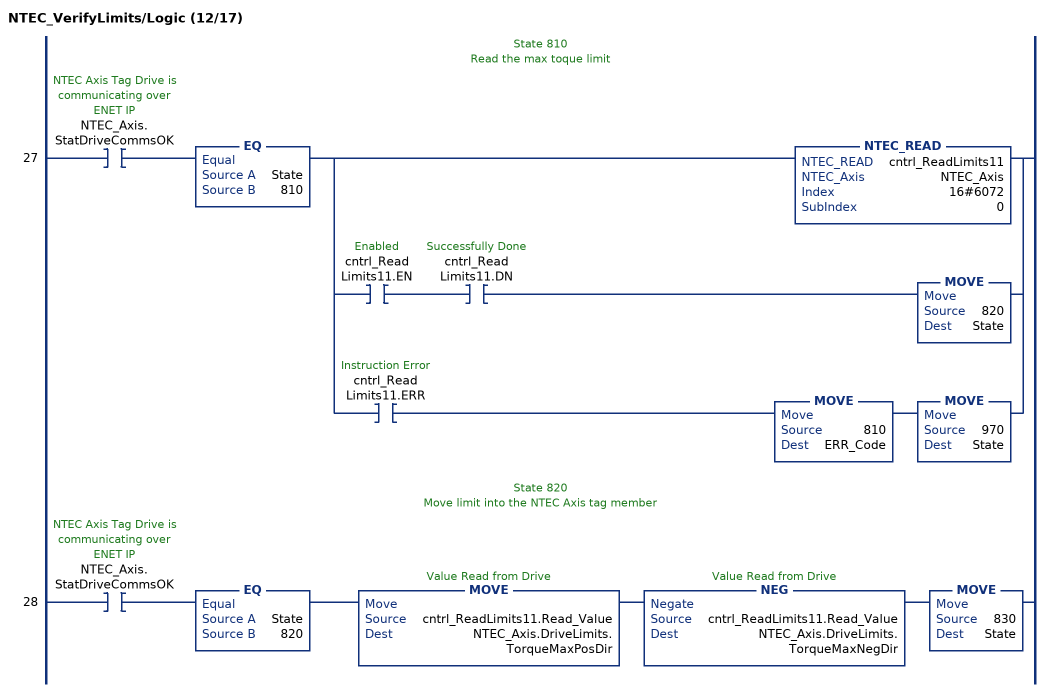
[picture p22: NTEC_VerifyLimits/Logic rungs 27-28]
   // State 810
   //   Read the max toque limit
   27: XIC(NTEC_Axis.StatDriveCommsOK)EQ(State,810)[NTEC_READ(cntrl_ReadLimits11,NTEC_Axis,16#6072,0) ,XIC(cntrl_ReadLimits11.EN) XIC(cntrl_ReadLimits11.DN) MOVE(820,State) ,XIC(cntrl_ReadLimits11.ERR) MOVE(810,ERR_Code) MOVE(970,State) ];
   // State 820
   // Move limit into the NTEC Axis tag member
   28: XIC(NTEC_Axis.StatDriveCommsOK)EQ(State,820)MOVE(cntrl_ReadLimits11.Read_Value,NTEC_Axis.DriveLimits.TorqueMaxPosDir)NEG(cntrl_ReadLimits11.Read_Value,NTEC_Axis.DriveLimits.TorqueMaxNegDir)MOVE(830,State);
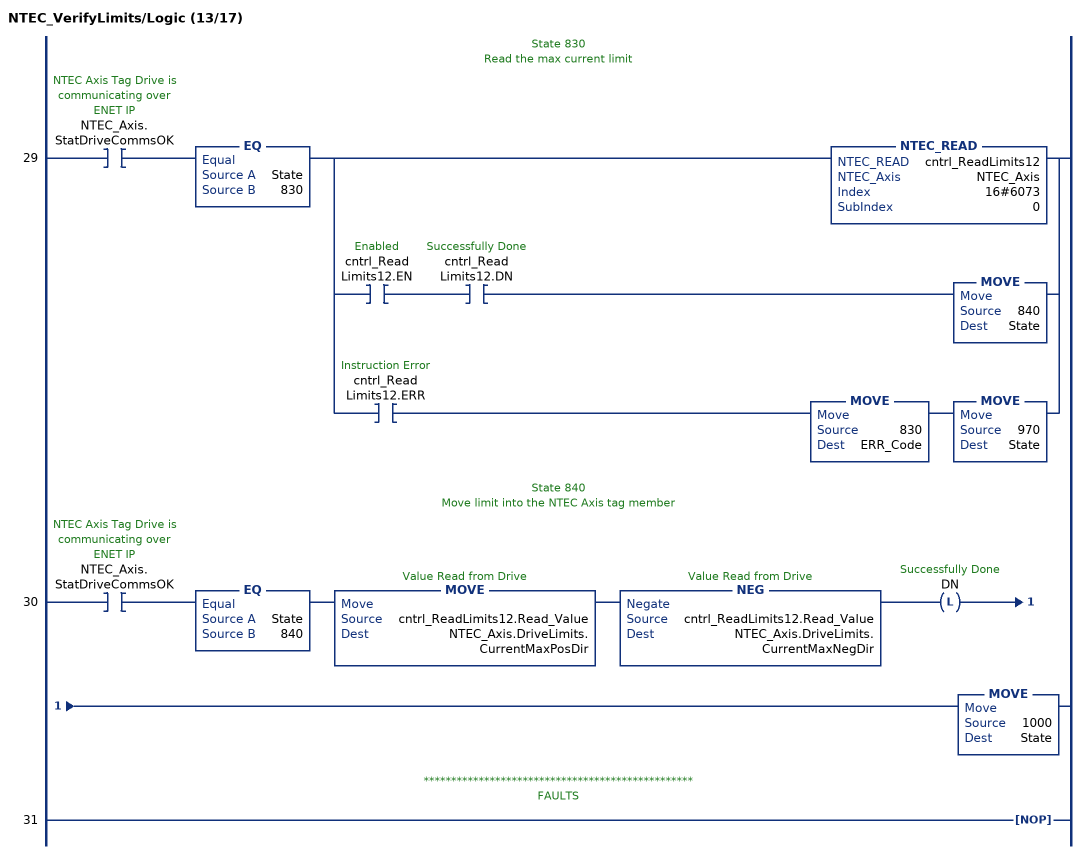
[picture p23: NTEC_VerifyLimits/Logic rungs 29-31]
   // State 830
   //   Read the max current limit
   29: XIC(NTEC_Axis.StatDriveCommsOK)EQ(State,830)[NTEC_READ(cntrl_ReadLimits12,NTEC_Axis,16#6073,0) ,XIC(cntrl_ReadLimits12.EN) XIC(cntrl_ReadLimits12.DN) MOVE(840,State) ,XIC(cntrl_ReadLimits12.ERR) MOVE(830,ERR_Code) MOVE(970,State) ];
   // State 840
   // Move limit into the NTEC Axis tag member
   30: XIC(NTEC_Axis.StatDriveCommsOK)EQ(State,840)MOVE(cntrl_ReadLimits12.Read_Value,NTEC_Axis.DriveLimits.CurrentMaxPosDir)NEG(cntrl_ReadLimits12.Read_Value,NTEC_Axis.DriveLimits.CurrentMaxNegDir)OTL(DN)MOVE(1000,State);
   // *************************************************
   // FAULTS
   31: NOP();
